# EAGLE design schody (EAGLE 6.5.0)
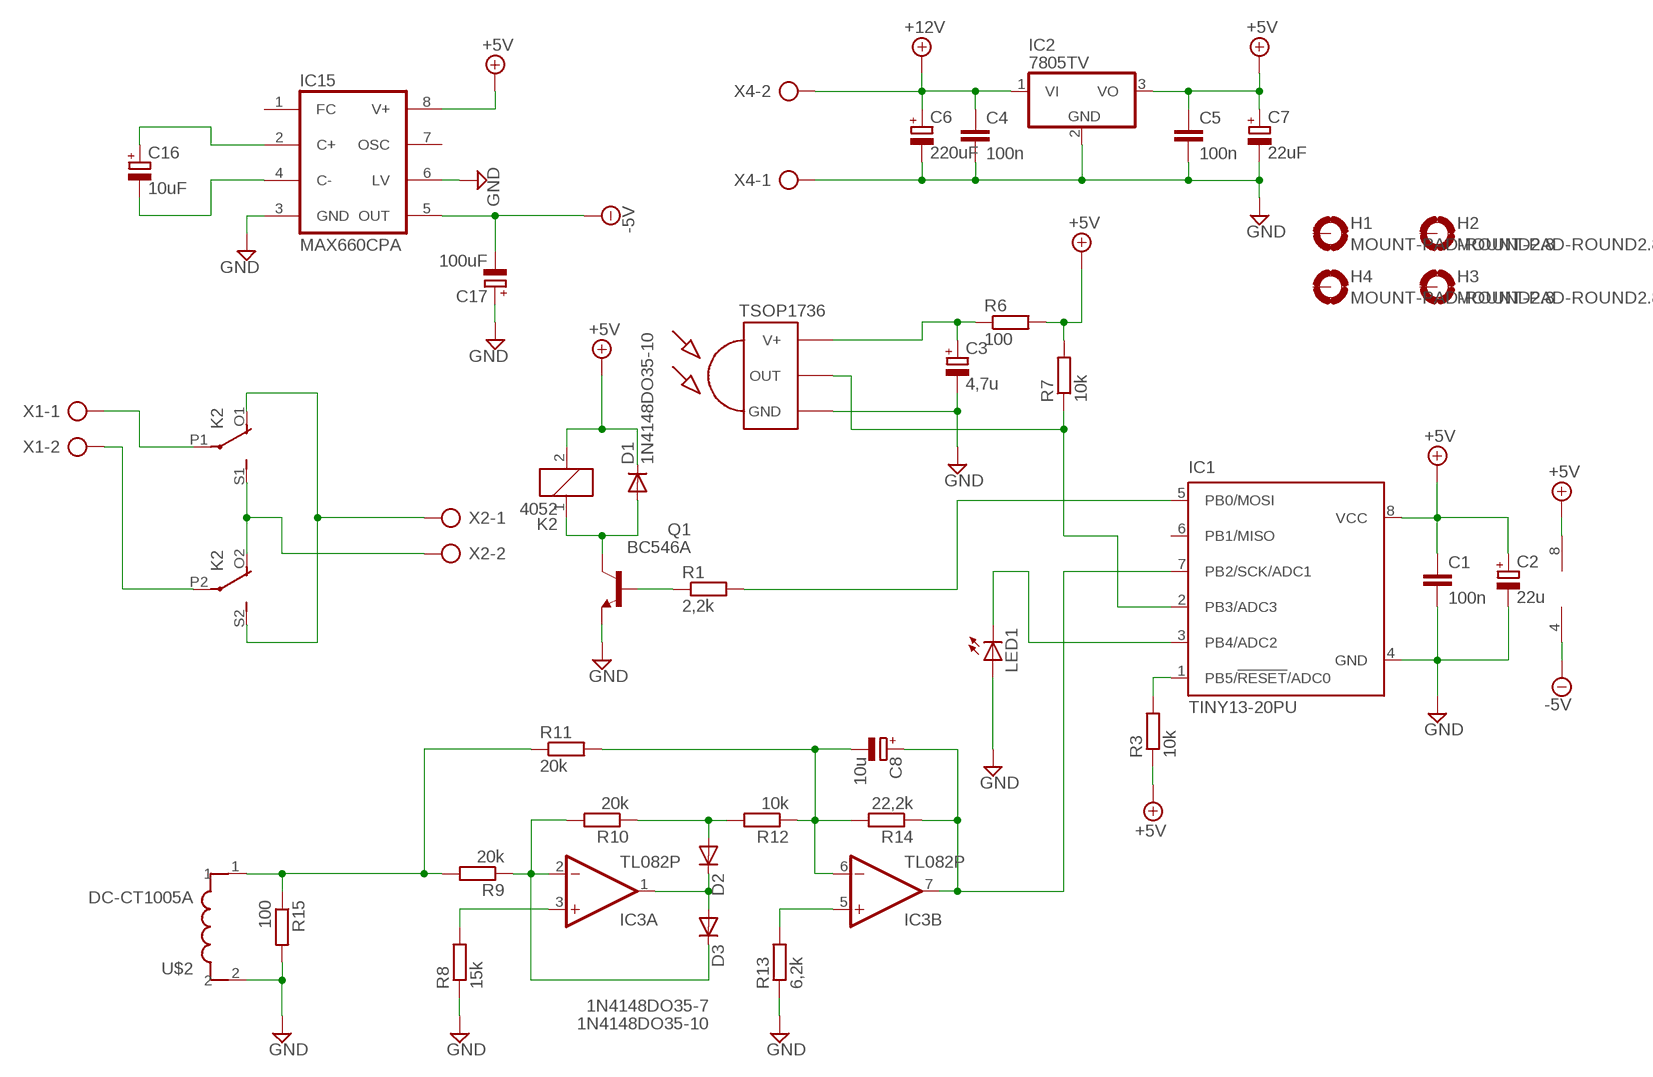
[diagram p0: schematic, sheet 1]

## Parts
C1  100n  C-EUC1206K  [C1206K]
C2  22u  CPOL-EUE2,5-6E  [E2,5-6E]
C3  4,7u  CPOL-EUE2,5-6E  [E2,5-6E]
C4  100n  C-EUC1206K  [C1206K]
C5  100n  C-EUC1206K  [C1206K]
C6  220uF  CPOL-EUE3.5-10  [E3,5-10]
C7  22uF  CPOL-EUE3.5-8  [E3,5-8]
C8  10u  CPOL-EUSMCD  [SMC_D]
C16  10uF  CPOL-EUE2.5-7  [E2,5-7]
C17  100uF  CPOL-EUE3.5-8  [E3,5-8]
D1  1N4148DO35-10  [DO35-10]
D2  1N4148DO35-10  [DO35-10]
D3  1N4148DO35-7  [DO35-7]
H1  MOUNT-PAD-ROUND2.8  [2,8-PAD]
H2  MOUNT-PAD-ROUND2.8  [2,8-PAD]
H3  MOUNT-PAD-ROUND2.8  [2,8-PAD]
H4  MOUNT-PAD-ROUND2.8  [2,8-PAD]
IC1  TINY13-20PU  [DIL08]
IC2  7805TV  [TO220V]
IC3  TL082P  [DIL08]
IC15  MAX660CPA  [DIL08]
K2  4052  [F4052]
LED1  LED5MM  [LED5MM]
Q1  BC546A  [TO92-EBC]
R1  2,2k  R-EU_R1206  [R1206]
R3  10k  R-EU_0204/7  [0204/7]
R6  100  R-EU_0207/10  [0207/10]
R7  10k  R-EU_0207/10  [0207/10]
R8  15k  R-EU_0204/7  [0204/7]
R9  20k  R-EU_0204/7  [0204/7]
R10  20k  R-EU_0204/7  [0204/7]
R11  20k  R-EU_0204/7  [0204/7]
R12  10k  R-EU_0207/10  [0207/10]
R13  6,2k  R-EU_0207/10  [0207/10]
R14  22,2k  R-EU_0204/7  [0204/7]
R15  100  R-EU_0204/7  [0204/7]
U$1  TSOP1736  [TSOP17XX]
U$2  DC-CT1005A  [DL-CT1005A]
X1  AK500/2  [AK500/2]
X2  AK500/2  [AK500/2]
X4  AK500/2  [AK500/2]

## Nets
+5V: C1.1 C2.+ C5.1 C7.+ D1.C IC1.8(VCC) IC2.3(VO) IC3.8(P:V+) IC15.8(V+) K2.2 R3.1 R6.2 R7.2
+12V: C4.1 C6.+ IC2.1(VI) X4.2
-5V: C17.- IC3.4(P:V-) IC15.5(OUT)
GND: C1.2 C2.- C3.- C4.2 C5.2 C6.- C7.- C17.+ IC1.4(GND) IC2.2(GND) IC15.3(GND) IC15.6(LV) LED1.A Q1.E R8.1 R13.1 R15.2 U$1.GND U$2.2 X4.1
N$1: C3.+ R6.1 U$1.V+
N$2: Q1.B R1.1
N$3: IC1.2(PB3/ADC3) R7.1 U$1.OUT
N$4: IC1.5(PB0/MOSI) R1.2
N$5: D1.A K2.1 Q1.C
N$6: IC1.3(PB4/ADC2) LED1.K(C)
N$9: K2.P1(2:P) X1.1
N$10: K2.P2(3:P) X1.2
N$11: K2.O1(2:O) K2.S2(3:S) X2.1
N$12: K2.O2(3:O) K2.S1(2:S) X2.2
N$13: D2.C D3.A IC3.1(A:OUT)
N$14: D3.C IC3.2(A:-IN) R9.1 R10.2
N$15: IC3.3(A:+IN) R8.2
N$16: IC1.1(PB5/!RESET!/ADC0) R3.2
N$17: R9.2 R11.1 R15.1 U$2.1
N$19: D2.A R10.1 R12.2
N$20: C8.- IC3.6(B:-IN) R11.2 R12.1 R14.2
N$21: IC3.5(B:+IN) R13.2
N$22: C8.+ IC1.7(PB2/SCK/ADC1) IC3.7(B:OUT) R14.1
N$96: C16.+ IC15.2(C+)
N$107: C16.- IC15.4(C-)
Unconnected: H1.B2,8(MOUNT) H2.B2,8(MOUNT) H3.B2,8(MOUNT) H4.B2,8(MOUNT) IC1.6(PB1/MISO) IC15.1(FC) IC15.7(OSC)

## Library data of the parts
C1 C4 C5 = rcl:C-EU: CAPACITOR, European symbol
C2 C3 C6-C8 C16 C17 = rcl:CPOL-EU: POLARIZED CAPACITOR, European symbol
D1-D3 = DIODY:1N4148: DIODE
H1-H4 = HOLES:MOUNT-PAD-ROUND: MOUNTING PAD, round
IC1 = atmega-atxmega:TINY13: 8-bit AVR Microcontroller with 1K Bytes In-System Programmable Flash Source: http://www.atmel.com/dyn/resources/prod_documents/2535S.pdf; MPN: ATTINY13-20PU; OC_FARNELL: 9171550; OC_NEWARK: 96K6521
IC2 = ANALOG:78*: Positive VOLTAGE REGULATOR Source: http://cache.national.com/ds/LM/LM78L05.pdf http://www.fairchildsemi.com/ds/LM/LM7805.pdf
IC3 = ANALOG:TL082: OP AMP
IC15 = maxim:MAX660CPA: Charge-pump VOLTAGE CONVERTER; MF: MAXIM; MPN: MAX660CPA; OC_FARNELL: 1187928; OC_NEWARK: 34C3964
K2 = PRZEKAŹNIKI:4052: RELAY 2 x switch, Finder; OC_FARNELL: unknown; OC_NEWARK: unknown
LED1 = led:LED: LED
Q1 = transistor-npn:BC546*: NPN Transistor
R1 R3 R6-R15 = rcl:R-EU_: RESISTOR, European symbol
U$1 = tsop-1:TSOP1736: IR Receiver and Demodulator
U$2 = MOJA:DC-CT1005A
X1 X2 X4 = ARK:AK500/2: CONNECTOR; OC_FARNELL: unknown; OC_NEWARK: unknown

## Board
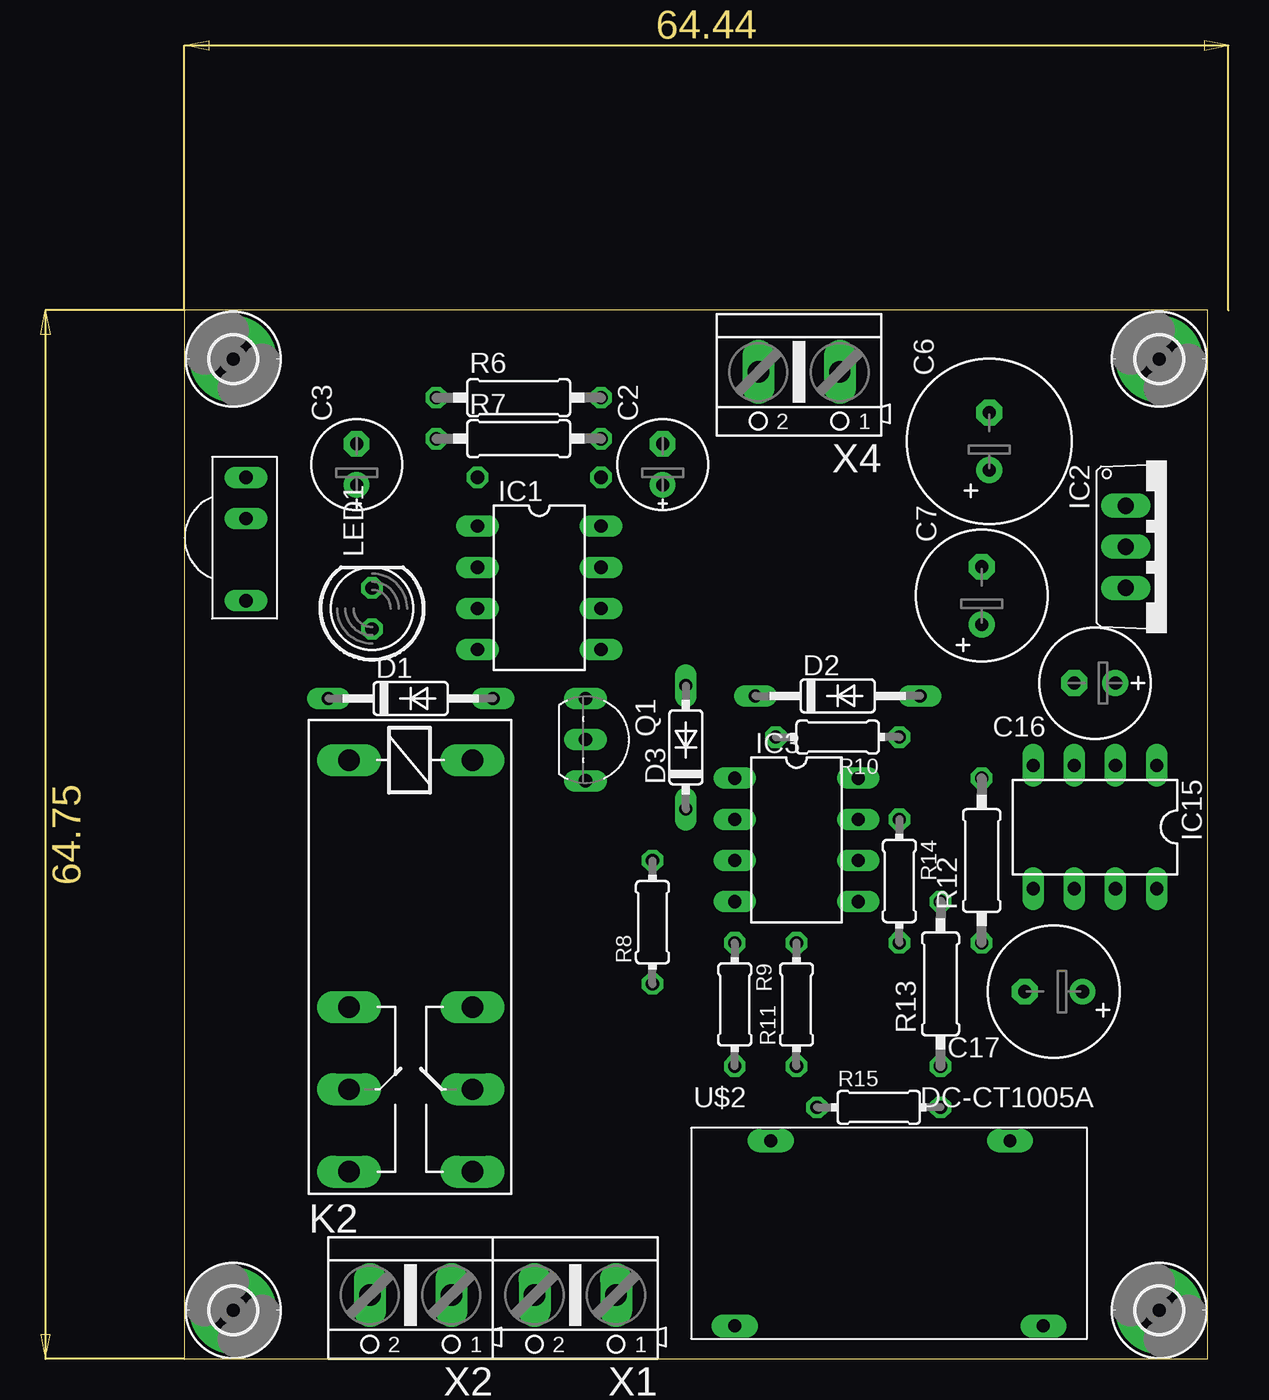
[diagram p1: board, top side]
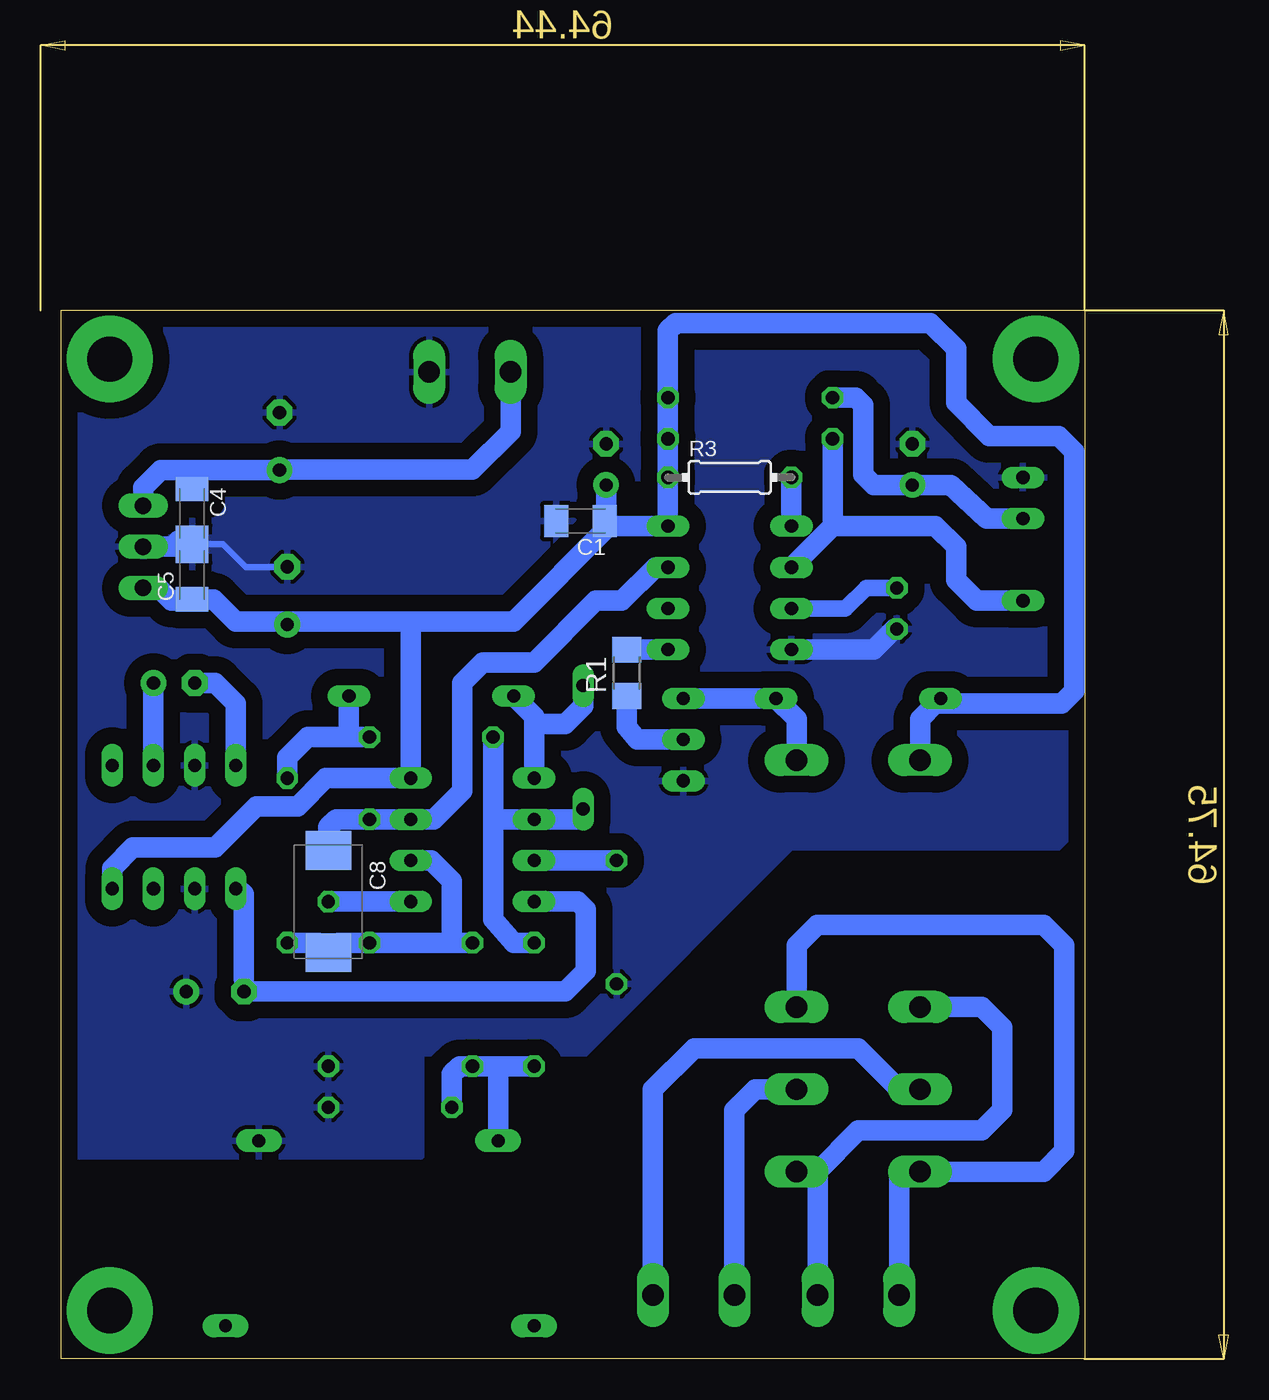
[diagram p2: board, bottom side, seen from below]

Size 73.31 x 81.4 mm. Coordinates in mm from the lower left corner, seen from the top.
Outline: 8.87,64.75 8.87,0 72.04,0 72.04,64.75 8.87,64.75
Copper layers (1*16): Top 0.035mm / dielectric 1.5mm / Bottom 0.035mm
Design rules "default": minimum track width 10mil, minimum drill 24mil, track to track 8mil, track to pad 8mil, pad to pad 8mil, via to via 8mil, smd to smd 8mil, copper to edge 40mil, drill to drill 8mil, minimum pad ring 10mil, minimum via ring 8mil, stop-mask expansion 4mil, vias tented up to drill 0mil, thermal gap 10mil

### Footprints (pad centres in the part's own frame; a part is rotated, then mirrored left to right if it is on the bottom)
C1206K = smd 1.5 x 2: 1 -1.5,0; 2 1.5,0
E2,5-6E = drill 0.813 pad 1.575: + -1.27,0 | drill 0.813 pad 1.575 octagon: - 1.27,0
E3,5-10 = drill 0.813 pad 1.6: + -1.778,0 | drill 0.813 pad 1.6 octagon: - 1.778,0
E3,5-8 = drill 0.813 pad 1.6: + -1.778,0 | drill 0.813 pad 1.6 octagon: - 1.778,0
SMC_D = smd 2.4 x 2.8: + -3.15,0; - 3.15,0
E2,5-7 = drill 0.813 pad 1.6: + -1.27,0 | drill 0.813 pad 1.6 octagon: - 1.27,0
DO35-10 = drill 0.813 long: A 5.08,0; C -5.08,0
DO35-7 = drill 0.813 long: A 3.81,0; C -3.81,0
2,8-PAD = drill 2.8 pad 5.334: B2,8 0,0
DIL08 = drill 0.813 long: 1 -3.81,-3.81; 2 -1.27,-3.81; 3 1.27,-3.81; 4 3.81,-3.81; 5 3.81,3.81; 6 1.27,3.81; 7 -1.27,3.81; 8 -3.81,3.81
TO220V = drill 1.016 long: 1 -2.54,-2.54; 2 0,-2.54; 3 2.54,-2.54
F4052 = drill 1.321 long: 1 -3.81,3.81; 2 -3.81,-3.81; O1 11.43,-3.81; O2 11.43,3.81; P1 16.51,-3.81; P2 16.51,3.81; S1 21.59,-3.81; S2 21.59,3.81
LED5MM = drill 0.813 octagon: A -1.27,0; K 1.27,0
TO92-EBC = drill 0.813 long: B 0,-1.27; C -2.54,-1.27; E 2.54,-1.27
R1206 = smd 1.6 x 1.803: 1 -1.422,0; 2 1.422,0
0204/7 = drill 0.813 octagon: 1 -3.81,0; 2 3.81,0
0207/10 = drill 0.813 octagon: 1 -5.08,0; 2 5.08,0
TSOP17XX = drill 0.813 long: GND -3.81,0; OUT 3.81,0; V+ -1.27,0
DL-CT1005A = drill 0.8 pad 1.422 long: 1 -7.938,5.556; 2 6.826,5.556; 3 8.89,-5.874; 4 -10.16,-5.874
AK500/2 = drill 1.321 long: 1 -2.515,0; 2 2.515,0

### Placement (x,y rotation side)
C1  39.99,51.73 180 bottom
C2  38.4,55.22 90 top
C3  19.51,55.22 90 top
C4  63.96,52.21 270 bottom
C5  63.96,48.4 90 bottom
C6  58.56,56.65 90 top
C7  58.09,47.13 90 top
C8  55.55,28.24 270 bottom
C16  65.07,41.73 180 top
C17  62.53,22.68 180 top
D1  22.84,40.78 0 top
D2  49.2,40.94 0 top
D3  39.83,37.76 90 top
H1  11.89,3 270 top
H2  11.89,61.73 270 top
H3  69.04,61.73 270 top
H4  69.04,3 270 top
IC1  30.78,47.6 270 top
IC2  69.52,50.14 270 top
IC3  46.66,32.05 270 top
IC15  65.07,32.84 180 top
K2  22.84,33.16 270 top
LED1  20.46,46.33 90 top
Q1  34.91,38.24 270 top
R1  37.13,42.37 90 bottom
R3  30.78,54.43 0 bottom
R6  29.51,59.35 0 top
R7  29.51,56.81 0 top
R8  37.77,26.97 90 top
R9  42.84,21.89 270 top
R10  49.2,38.4 180 top
R11  46.66,21.89 90 top
R12  58.09,30.78 90 top
R13  55.55,23.16 90 top
R14  53,29.51 270 top
R15  51.73,15.54 0 top
U$1  12.68,50.62 270 top
U$2  53,7.92 0 top
X1  33,3.95 180 top
X2  22.84,3.95 180 top
X4  46.81,60.94 180 top

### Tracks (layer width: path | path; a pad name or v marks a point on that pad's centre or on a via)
+5V
  Bottom 1.27: 38.24,51.42 38.4,51.42 38.4,51.89 | 38.24,51.42 IC1.8 R3.1 R7.2 R6.2 34.59,63.48 34.11,63.96 18.4,63.96 16.81,62.37 16.81,59.04 14.75,56.97 10.46,56.97 9.51,56.02 9.51,41.26 10.3,40.46 18.08,40.46 | C2.+ 38.4,51.89 | IC15.8 68.88,30.3 67.61,31.57 62.53,31.57 59.99,34.11 57.45,34.11 55.7,35.86 IC3.8 50.47,45.54 | 38.24,51.42 44.12,45.54 50.47,45.54 | 50.47,45.54 57.89,45.54 C7.+ 58.28,45.54 61.26,45.54 62.62,46.9 C5.1 64.05,46.81 65.23,46.81 66.02,47.61 IC2.3 | C1.1 38.49,51.98 38.4,51.89 | K2.2 19.03,39.51 18.08,40.46 | 18.08,40.46 D1.C
+12V
  Bottom 1.27: 63.86,53.61 C4.1 63.96,54.88 | 63.96,54.88 C6.+ 58.53,54.91 46.66,54.91 44.3,57.26 X4.2 | 63.96,54.88 65.9,54.88 66.97,53.8 IC2.1
-5V
  Bottom 1.27: IC15.5 61.1,29.03 60.78,28.71 60.78,23.98 C17.- | 60.78,23.92 C17.- | IC3.4 40.15,28.24 39.67,27.76 39.67,23.95 40.94,22.68 C17.-
GND
  Bottom 0.406: C7.- 60.66,48.91 62.05,50.3 63.55,50.3 C4.2
  Bottom 1.27: C4.2 C5.2 | LED1.A 20.62,45.07 21.89,43.8 IC1.4 | IC2.2 64.2,50.15 C5.2 | C5.2 64.82,50.53 63.64,50.62
  pour Bottom (isolate 1.016): 7.92,65.86 72.69,65.86 72.69,12.52 49.83,12.52 49.83,18.87 39.67,18.87 26.97,31.57 10.46,31.57 7.92,34.11
N$1
  Bottom 1.27: R6.1 23,59.35 22.52,58.88 22.52,54.59 21.89,53.96 C3.+ 17.13,53.96 14.91,51.89 U$1.V+
N$2
  Bottom 1.27: Q1.B 36.49,38.24 37.13,39.03 R1.1
N$3
  Bottom 1.27: 24.43,51.42 18.08,51.42 16.81,50.15 16.81,48.08 15.54,46.81 U$1.OUT | 24.43,51.42 IC1.2 | R7.1 24.43,51.42
N$4
  Bottom 1.27: R1.2 IC1.5
N$5
  Bottom 1.27: K2.1 26.65,39.51 D1.A Q1.C
N$6
  Bottom 1.016: IC1.3 23.64,46.34 22.37,47.61 LED1.K
N$9
  Bottom 1.27: X1.1 35.52,16.65 32.98,19.19 22.84,19.19 20.3,16.65 K2.P1
N$10
  Bottom 1.27: X1.2 30.49,15.35 29.19,16.65 K2.P2
N$11
  Bottom 1.27: X2.1 25.36,11.54 K2.S2 25.38,11.57 22.84,14.11 15.22,14.11 13.95,15.38 13.95,20.46 15.22,21.73 K2.O1
N$12
  Bottom 1.27: X2.2 20.33,11.54 K2.S1 11.41,11.57 10.14,12.84 10.14,25.54 11.41,26.81 25.38,26.81 26.65,25.54 K2.O2
N$13
  Bottom 1.27: 42.84,39.19 42.84,39.67 D2.C | 42.84,39.19 IC3.1 | D3.A 39.83,40.3 40.94,39.19 42.84,39.19
N$14
  Bottom 1.27: 45.38,33.32 45.38,27.13 44.12,25.7 R9.1 | 45.38,33.32 IC3.2 39.83,33.32 D3.C | R10.2 45.38,33.32
N$15
  Bottom 1.27: IC3.3 R8.2
N$16
  Bottom 1.27: R3.2 IC1.1
N$17
  Bottom 1.27: U$2.1 45.07,18.08 | 45.07,18.08 R11.1 47.45,18.08 47.92,17.6 R15.1 | 45.07,18.08 R9.2
N$19
  Bottom 1.27: R12.2 58.09,37.13 56.81,38.4 54.27,38.4 | 54.27,38.4 R10.1 | D2.A 54.27,38.4
N$20
  Bottom 1.27: R11.2 47.92,25.7 | 47.92,25.7 47.92,29.51 49.2,30.78 IC3.6 | 47.92,25.7 R14.2 54.94,25.7 C8.- 56.16,25.7 R12.1
N$21
  Bottom 1.27: IC3.5 R13.2
N$22
  Bottom 1.27: C8.+ 55.55,32.84 55.07,33.32 R14.1 IC3.7 49.04,33.32 47.29,35.06 47.29,41.73 46.02,43 42.84,43 39.03,46.81 37.45,46.81 35.38,48.88 IC1.7
N$96
  Bottom 1.27: IC15.2 C16.+
N$107
  Bottom 1.27: C16.- 62.53,41.73 61.26,40.46 IC15.4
